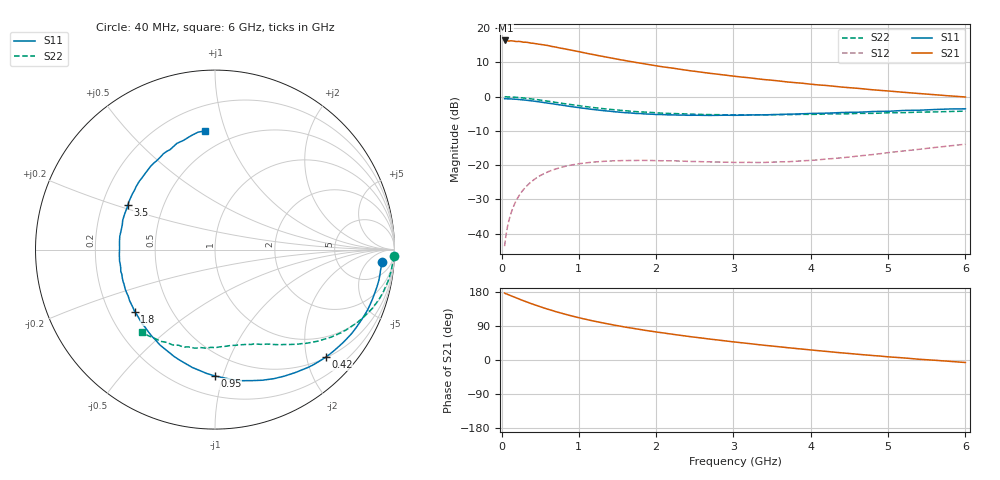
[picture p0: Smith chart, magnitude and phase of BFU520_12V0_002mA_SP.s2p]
! Filename:  P:\Prog\Test\Noise\ATS_data\Testdata_Net\03 Spar\BFU520_APG2013_37_A05_12p0V_002mA_SP_CM01_D.s2p
! Date/Time: Fri 26/Apr/2013 13:00:11
! BFU520_APG2013_37_A05_12p0V_1to20mA_SP_CM01_Bias2_R.s2p
! MDIF S-parameter v. bias file
! BFU520_APG2013_37_A05_12p0V_1to20mA_SP_CM01
! Date/time Tue Apr 23 18:22:57 2013
! VAR V_out= 12.0000
! VAR I_out= 2.0050
! VAR V_in= 0.8006
! VAR I_in= 0.0179
! Device data file deembeded for feedlines and parallel
! Original file: \03 Spar\BFU520_APG2013_37_A05_12p0V_002mA_SP_CM01_R.s2p
! Feed-files: PR047V01_250413_Feed1.s2p, PR047V01_250413_Feed2.s2p
! Parallel-file: PR047V01_250413_Par.s2p
# MHz S MA R 50
!  Freq-MHz  S11-mag  S11-arg  S21-mag  S21-arg  S12-mag  S12-arg  S22-mag  S22-arg
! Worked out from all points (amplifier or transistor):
!   98 points, 40 MHz to 6 GHz, reference 50 ohm
!   highest |S21| = 16.4 dB at 50 MHz (marker M1)
!   |S21| within 3 dB of that: start of sweep to 941 MHz
!   unconditionally stable (mu >= 1): 3.033 GHz to 4.918 GHz
!   at 300 MHz: K = 0.11, MSG = 21.3 dB, |S12| = -26.7 dB
!   at 1.6 GHz: K = 0.52, MSG = 14.6 dB, |S12| = -18.7 dB
!   at 6 GHz: K = 0.82, MSG = 6.9 dB, |S12| = -13.9 dB
!   S11 on the Smith chart (normalised r, x): 40 MHz: 13, -14; 420 MHz: 0.52, -2.37; 950 MHz: 0.34, -0.94; 1.8 GHz: 0.31, -0.31; 3.5 GHz: 0.31, +0.22; 6 GHz: 0.36, +0.85
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40  0.9328 -4.3  6.609 176.7  0.006535 85.8  0.9954 -2.0
50  0.9317 -5.4  6.625 175.1  0.008192 85.2  0.9979 -2.7
100  0.9288 -10.7  6.501 171.5  0.01619 82.6  0.9903 -5.8
120  0.9259 -13.0  6.557 169.7  0.01937 81.4  0.9881 -7.0
180  0.917 -19.4  6.42 164.9  0.02876 77.5  0.9797 -10.5
240  0.9049 -25.8  6.393 159.9  0.03766 73.8  0.9675 -13.9
320  0.8864 -34.1  6.238 153.6  0.04877 68.9  0.9469 -18.4
420  0.8599 -44.1  6.004 146.2  0.06126 63.2  0.9164 -23.3
550  0.8187 -56.7  5.696 137.2  0.07495 56.3  0.8733 -29.3
700  0.774 -70.1  5.305 127.8  0.08764 49.5  0.8252 -35.2
950  0.7035 -90.2  4.669 114.1  0.1023 40.4  0.7503 -43.3
1050  0.6784 -97.4  4.423 109.2  0.1063 37.4  0.7246 -46.2
1200  0.6461 -107.8  4.093 102.4  0.1109 33.4  0.6905 -49.9
1450  0.6028 -123.3  3.616 92.4  0.1154 28.2  0.6452 -55.2
1800  0.5661 -142.1  3.082 80.3  0.1169 23.2  0.599 -61.5
2050  0.548 -154.1  2.766 72.6  0.1158 21.0  0.5761 -65.9
2450  0.5343 -171.7  2.383 61.4  0.1129 19.3  0.5537 -72.5
3100  0.5349 164.8  1.937 45.6  0.1093 22.3  0.5417 -82.6
3500  0.5459 152.8  1.737 36.8  0.1105 26.3  0.5451 -88.9
4100  0.5706 135.3  1.484 24.6  0.1194 33.0  0.5525 -98.9
5200  0.6289 109.7  1.158 5.5  0.1608 39.4  0.5829 -117.5
6000  0.6641 94.7  0.989 -6.6  0.202 37.5  0.6138 -131.4
